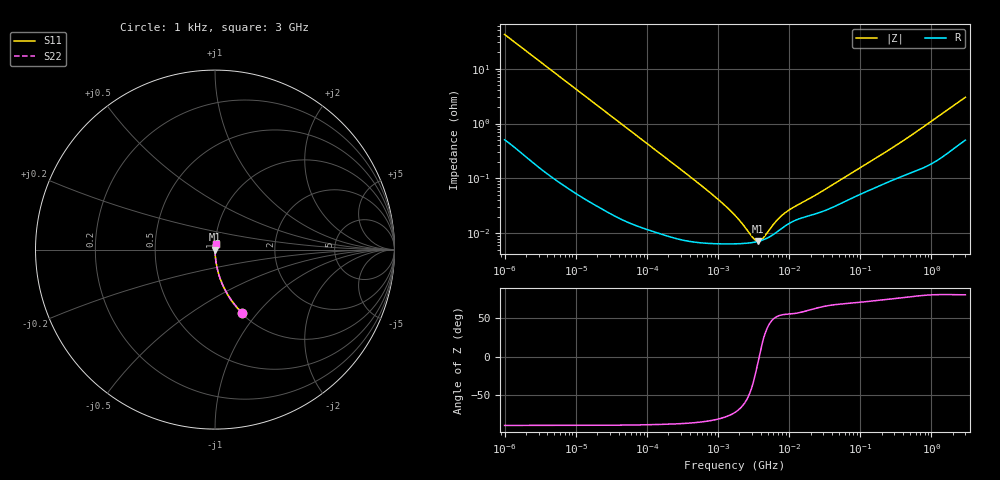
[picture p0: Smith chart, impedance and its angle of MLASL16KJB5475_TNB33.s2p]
! MLASL16KJB5475_TNB33  S-PARAMETER MODEL  ( Standard Model )
! Model Generated by TAIYO YUDEN Corporation (http://www.ty-top.com)
! Version 1.0
! TAIYO YUDEN Control No. 220601
! Copyright(c) 2012 TAIYO YUDEN CO.,LTD. All Rights Reserved.
! Product Description (link to TY-COMPAS)
! https://ds.yuden.co.jp/TYCOMPAS/or/detail?pn=MLASL16KJB5475MTNB33&u=M
! Products Name : Multilayer Ceramic Capacitors
! Characteristics :
!  Capacitance : 4.7 [uF] , Rated Voltage : 10 [V] , TCC : X5R
!  Case Size : 1.6 x 0.8 / 0.063 x 0.031 [mm/inch] , Thickness : 0.45 / 0.018 [mm/inch]
!  (Conditions: Temperature = 25 [degC] , DC Bias Voltage = 0 [V])
! External Node Assignments :
!  1  o---| |---o  2
! GND o---------o GND
! Frequency Range : 1kHz  -  3GHz  [ 401 STEP ]
# MHZ S RI R 50
! Freq[MHz].  S11 Real  S11 Imag  S21 Real  S21 Imag  S12 Real  S12 Imag  S22 Real  S22 Imag
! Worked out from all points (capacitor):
!   401 points, 1 kHz to 3 GHz, reference 50 ohm
!   read as one part in series: C = 3.79 uF near 1.077 kHz
!   lowest |Z| = 7.15 mohm at 3.651 MHz (marker M1)
!   series resonance near 3.783 MHz, so ESL is about 470 pH
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0.001  0.1525 -0.3535  0.8475 0.3535  0.8475 0.3535  0.1525 -0.3535
0.001685  0.0612 -0.2339  0.9388 0.2339  0.9388 0.2339  0.0612 -0.2339
0.003177  0.0189 -0.1305  0.9811 0.1305  0.9811 0.1305  0.0189 -0.1305
0.005768  0.00623 -0.0731  0.9938 0.0731  0.9938 0.0731  0.00623 -0.0731
0.01216  0.00168 -0.035  0.9983 0.035  0.9983 0.035  0.00168 -0.035
0.147855  0.000108 -0.00294  0.9999 0.00294  0.9999 0.00294  0.000108 -0.00294
0.762639  6.54e-05 -0.000554  0.9999 0.000554  0.9999 0.000554  6.54e-05 -0.000554
1.238299  6.41e-05 -0.000318  0.9999 0.000318  0.9999 0.000318  6.41e-05 -0.000318
1.732051  6.42e-05 -0.000202  0.9999 0.000202  0.9999 0.000202  6.42e-05 -0.000202
2.709407  6.64e-05 -8e-05  0.9999 8e-05  0.9999 8e-05  6.64e-05 -8e-05
2.919173  6.72e-05 -6.18e-05  0.9999 6.18e-05  0.9999 6.18e-05  6.72e-05 -6.18e-05
3.651041  7.1e-05 -8.36e-06  0.9999 8.36e-06  0.9999 8.36e-06  7.1e-05 -8.36e-06
4.739869  7.99e-05 5.34e-05  0.9999 -5.34e-05  0.9999 -5.34e-05  7.99e-05 5.34e-05
5.106836  8.38e-05 7.12e-05  0.9999 -7.12e-05  0.9999 -7.12e-05  8.38e-05 7.12e-05
6.881678  0.000108 0.000141  0.9999 -0.000141  0.9999 -0.000141  0.000108 0.000141
8.606987  0.000133 0.00019  0.9999 -0.00019  0.9999 -0.00019  0.000133 0.00019
11.1738  0.000163 0.000241  0.9998 -0.000241  0.9998 -0.000241  0.000163 0.000241
21.06097  0.000217 0.000401  0.9998 -0.000401  0.9998 -0.000401  0.000217 0.000401
256.0921  0.000886 0.00321  0.9991 -0.00321  0.9991 -0.00321  0.000886 0.00321
520.0673  0.0013 0.00595  0.9987 -0.00595  0.9987 -0.00595  0.0013 0.00595
2144.796  0.00409 0.0218  0.9959 -0.0218  0.9959 -0.0218  0.00409 0.0218
3000  0.00582 0.0292  0.9942 -0.0292  0.9942 -0.0292  0.00582 0.0292
